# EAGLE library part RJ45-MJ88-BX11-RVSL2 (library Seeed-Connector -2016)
320140004
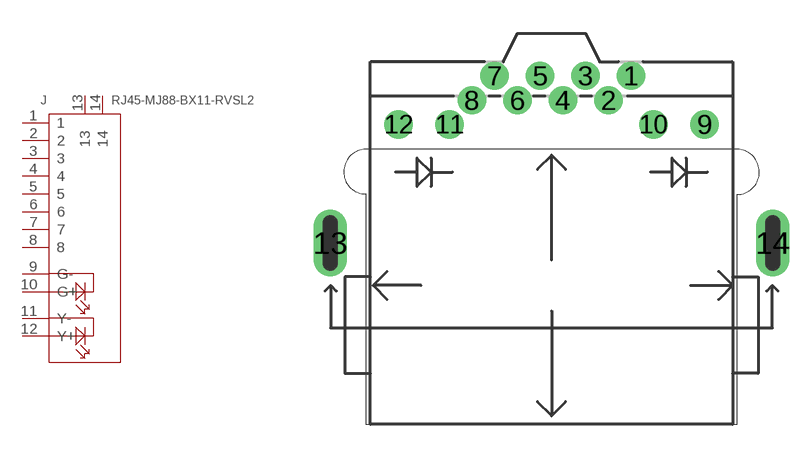
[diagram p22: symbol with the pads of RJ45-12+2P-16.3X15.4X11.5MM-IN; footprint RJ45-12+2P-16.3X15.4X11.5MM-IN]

Designator prefix J

## RJ45-MJ88-BX11-RVSL2 (MPN: MJ88-BX11-RVSL2; VALUE: MJ88-BX11-RVSL2)  [RJ45-12+2P-16.3X15.4X11.5MM-IN]
1  1
2  2
3  3
4  4
5  5
6  6
7  7
8  8
9  G-
10  G+
11  Y-
12  Y+
13  13
14  14

## Footprint RJ45-12+2P-16.3X15.4X11.5MM-IN (pad centres in mm)
drill 0.762 pad 1.27: 1 3.57,7.5; 2 2.55,6.4; 3 1.53,7.5; 4 0.51,6.4; 5 -0.51,7.5; 6 -1.53,6.4; 7 -2.55,7.5; 8 -3.57,6.4; 9 6.86,5.32; 10 4.57,5.32; 11 -4.57,5.32; 12 -6.86,5.32
drill 0.6 pad 1.5 long: 13 -9.92,0; 14 9.92,0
